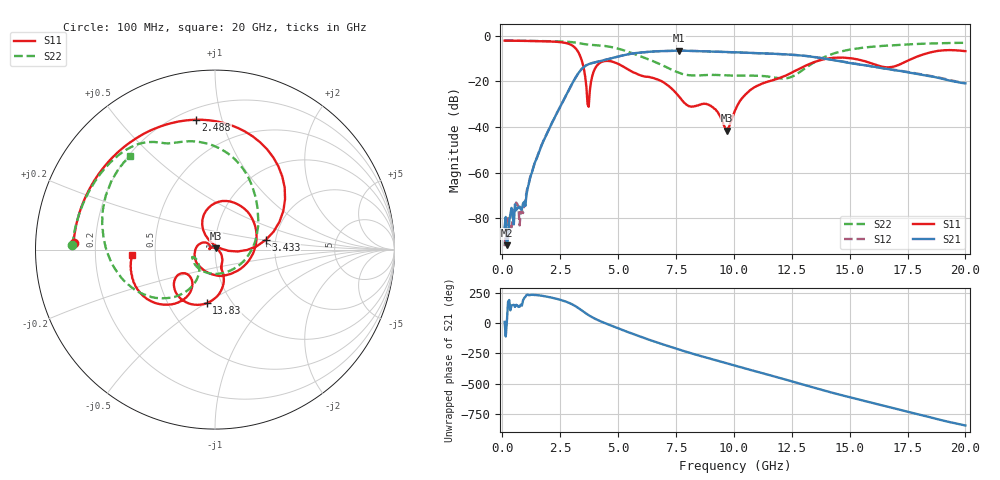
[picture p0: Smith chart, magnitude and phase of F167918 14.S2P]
!  2-Port S-parameters saved by WinCal
! VAR MeasName=S-Parameters (CALIBRATED_DATA) read from VNA (N5242A)
! VAR MeasDate=2016-11-22 10:25:28
! VAR NAME=F167918 14
! VAR FILENAME=F167918 14.S2P
! VAR DATE=2016-11-22 10:25:28
! VAR PHYS_PORTS=1,2
# Hz S DB R 50
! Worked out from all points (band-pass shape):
!   401 points, 100 MHz to 20 GHz, reference 50 ohm
!   highest |S21| = -6.49 dB at 7.612 GHz (marker M1); lowest = -91.9 dB at 199.5 MHz (marker M2)
!   |S21| within 3 dB of the highest: 4.835 GHz to 13.62 GHz (8.786 GHz wide, 95.2 % of centre)
!   lowest |S11| = -41.6 dB at 9.702 GHz (marker M3), VSWR 1.02, Z = 50.3 + j0.779 ohm
!   |S11| at or under -10 dB: 3.405 GHz to 14.02 GHz (10.61 GHz wide, 122 % of centre); 15.18 GHz to 17.71 GHz (2.53 GHz wide, 15.4 % of centre)
!   |S22| runs from -18.7 to -2.0 dB; largest |S21 - S12| = 0.0041
!   S11 on the Smith chart (normalised r, x): 100 MHz: 0.12, +0.02; 2.488 GHz: 0.27, +0.83; 3.433 GHz: 1.77, +0.21; 13.83 GHz: 0.77, -0.50; 20 GHz: 0.37, -0.03
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1e8  -2.07 177.3  -83.83 11.5  -92.25 171.3  -2.00 178.3
1.995e8  -2.07 174.6  -91.89 18.4  -88.01 119.1  -2.01 176.7
8.4625e8  -2.18 157.3  -76.09 145.8  -76.57 -172.7  -2.12 166.5
1.493e9  -2.29 138.5  -53.65 -127.9  -53.16 -128.4  -2.22 156.2
2.488e9  -2.72 98.3  -31.30 -165.1  -31.33 -165.5  -2.42 138.4
3.13475e9  -5.14 47.4  -18.81 144.0  -18.84 143.9  -2.90 123.9
3.43325e9  -10.83 10.7  -14.48 105.8  -14.47 105.8  -3.43 117.6
3.73175e9  -31.10 101.7  -12.39 66.5  -12.37 66.4  -3.83 112.9
3.9805e9  -14.80 112.6  -11.66 39.8  -11.63 39.5  -4.00 108.2
4.3785e9  -11.11 76.6  -10.71 5.4  -10.71 5.0  -4.35 98.2
5.672e9  -16.06 -62.6  -7.66 -90.7  -7.65 -90.7  -7.82 59.1
6.7665e9  -19.35 177.3  -6.70 -164.0  -6.71 -164.2  -12.22 18.6
7.61225e9  -26.32 139.0  -6.49 144.0  -6.52 143.9  -16.11 -37.0
9.00525e9  -30.64 163.0  -6.85 65.0  -6.84 64.8  -17.12 -133.7
9.70175e9  -41.56 67.8  -7.08 27.6  -7.09 27.6  -17.29 -153.3
1.005e10  -32.74 -16.2  -7.19 9.2  -7.21 9.3  -17.47 -157.4
1.17415e10  -19.28 -71.4  -7.86 -79.5  -7.85 -79.3  -18.21 -158.8
1.338325e10  -11.84 -86.4  -9.13 -168.5  -9.09 -168.1  -12.14 -122.4
1.3831e10  -10.38 -98.9  -9.84 167.5  -9.76 167.8  -9.62 -128.8
1.67165e10  -13.80 -132.9  -14.61 26.6  -14.58 26.8  -4.21 176.3
1.845775e10  -7.32 -135.0  -17.72 -56.2  -17.51 -56.8  -3.33 152.1
2e10  -6.68 -176.2  -20.83 -124.8  -20.73 -125.6  -3.05 132.0
